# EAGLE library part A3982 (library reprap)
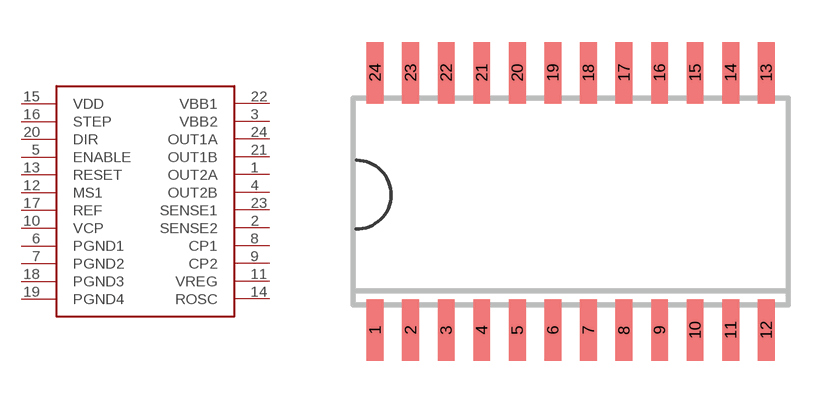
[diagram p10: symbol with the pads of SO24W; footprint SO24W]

Designator prefix -

## A3982SOIC24  [SO24W]
1  OUT2A
2  SENSE2
3  VBB2
4  OUT2B
5  ENABLE
6  PGND1
7  PGND2
8  CP1
9  CP2
10  VCP
11  VREG
12  MS1
13  RESET
14  ROSC
15  VDD
16  STEP
17  REF
18  PGND3
19  PGND4
20  DIR
21  OUT1B
22  VBB1
23  SENSE1
24  OUT1A

## Footprint SO24W (pad centres in mm)
SMALL OUTLINE INTEGRATED CIRCUIT wide body 7.5 mm/JEDEC MO-119AA
smd 0.6 x 2.2: 1 -6.985,-4.6; 2 -5.715,-4.6; 3 -4.445,-4.6; 4 -3.175,-4.6; 5 -1.905,-4.6; 6 -0.635,-4.6; 7 0.635,-4.6; 8 1.905,-4.6; 9 3.175,-4.6; 10 4.445,-4.6; 11 5.715,-4.6; 12 6.985,-4.6; 13 6.985,4.6; 14 5.715,4.6; 15 4.445,4.6; 16 3.175,4.6; 17 1.905,4.6; 18 0.635,4.6; 19 -0.635,4.6; 20 -1.905,4.6; 21 -3.175,4.6; 22 -4.445,4.6; 23 -5.715,4.6; 24 -6.985,4.6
